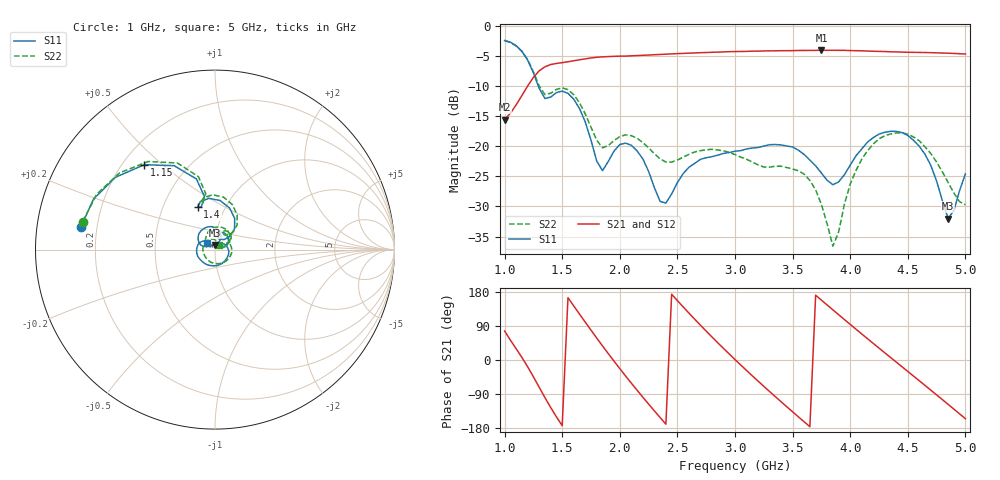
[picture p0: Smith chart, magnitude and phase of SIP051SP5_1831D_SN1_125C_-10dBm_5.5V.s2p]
# GHz  S  dB  R  50
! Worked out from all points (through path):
!   81 points, 1 GHz to 5 GHz, reference 50 ohm
!   highest |S21| = -4.04 dB at 3.75 GHz (marker M1); lowest = -15.6 dB at 1 GHz (marker M2)
!   lowest |S11| = -32.0 dB at 4.85 GHz (marker M3), VSWR 1.05, Z = 49.9 + j2.5 ohm
!   |S11| at or under -10 dB: 1.293 GHz to end of sweep
!   |S22| runs from -36.6 to -2.5 dB; largest |S21 - S12| = 0.0019
!   S11 on the Smith chart (normalised r, x): 1 GHz: 0.14, +0.08; 1.15 GHz: 0.29, +0.44; 1.4 GHz: 0.74, +0.38; 5 GHz: 0.91, +0.07
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1  -2.41 170.3  -15.57 76.7  -15.59 76.8  -2.46 168.0
1.15  -4.21 129.8  -11.57 6.7  -11.57 6.7  -4.21 127.2
1.25  -7.80 104.8  -8.55 -44.2  -8.55 -44.2  -7.61 102.8
1.4  -11.82 112.1  -6.41 -125.4  -6.41 -125.5  -11.18 107.1
1.55  -11.20 84.4  -5.95 164.5  -5.94 164.4  -10.59 80.6
1.7  -15.95 46.9  -5.47 100.0  -5.45 100.0  -14.62 48.4
1.85  -24.05 68.4  -5.14 37.1  -5.14 37.2  -20.26 56.6
1.95  -20.79 78.7  -5.05 -3.2  -5.05 -3.2  -19.05 65.6
2.15  -20.77 34.6  -4.92 -79.7  -4.91 -79.7  -18.66 39.3
2.35  -29.16 21.7  -4.74 -151.9  -4.73 -151.8  -22.08 27.0
2.5  -26.03 40.5  -4.60 156.7  -4.59 156.7  -22.30 28.6
2.7  -22.17 -6.8  -4.44 91.9  -4.43 91.8  -20.73 9.6
3  -20.82 -91.5  -4.26 1.2  -4.26 1.2  -21.38 -60.1
3.35  -19.71 -168.9  -4.13 -96.7  -4.13 -96.7  -23.32 174.1
3.7  -23.26 137.0  -4.06 171.0  -4.06 170.9  -27.23 78.4
3.75  -24.44 136.5  -4.04 158.0  -4.05 158.0  -29.66 74.1
3.85  -26.39 147.8  -4.04 132.3  -4.03 132.3  -36.60 100.1
4.05  -21.59 162.5  -4.11 81.4  -4.11 81.4  -24.04 140.8
4.35  -17.52 117.0  -4.30 6.7  -4.31 6.7  -17.96 84.4
4.65  -21.35 66.8  -4.42 -67.2  -4.43 -67.3  -20.11 32.6
4.85  -32.01 91.5  -4.53 -117.1  -4.54 -117.0  -26.01 20.8
5  -24.60 140.1  -4.66 -154.9  -4.67 -154.9  -29.71 53.1
